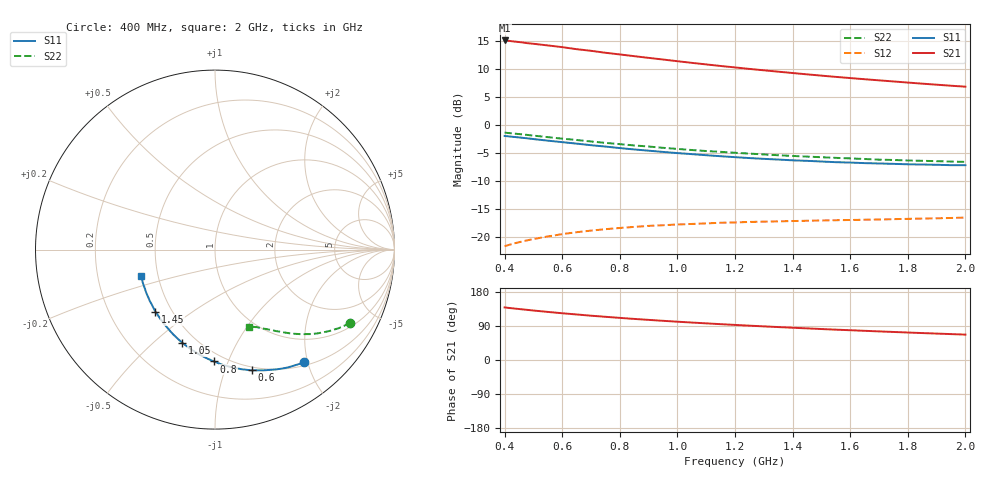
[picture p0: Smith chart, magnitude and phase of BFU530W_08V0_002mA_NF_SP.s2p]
! Filename:  P:\Prog\Test\Noise\ATS_data\Testdata_Net\06 Compressed Noise after Statistics\BFU530W_APM2013_09_A05_08p0V_002mA_NF_CM01_D.sf
! Date/Time: Tue 26/Mar/2013 18:06:04
! BFU530W_APM2013_09_A05_08p0V_1to25mA_NF_CM01_Bias2_R.sf
! Noise Parameter Data File
! BFU530W_APM2013_09_A05_08p0V_1to25mA_NF_CM01
! Date/time: Thu Mar 21 21:44:48 2013
! VAR V_out= 8.000000
! VAR I_out= 2.000000
! VAR V_in= 0.795400
! VAR I_in= 0.019805
! Device data file deembeded for feedlines and parallel
! Original file: \06 Compressed Noise after Statistics\BFU530W_APM2013_09_A05_08p0V_002mA_NF_CM01_R.sf
! Feed-files: PR019V01_070313_Feed1.s2p, PR019V01_070313_Feed2.s2p
! Parallel-file: PR019V01_070313_Par.s2p
# MHz S MA R 50
!  Freq-MHz  S11-mag  S11-arg  S21-mag  S21-arg  S12-mag  S12-arg  S22-mag  S22-arg
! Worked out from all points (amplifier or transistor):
!   37 points, 400 MHz to 2 GHz, reference 50 ohm
!   highest |S21| = 15.1 dB at 400 MHz (marker M1)
!   |S21| within 3 dB of that: start of sweep to 882.4 MHz
!   unconditionally stable (mu >= 1): nowhere
!   at 500 MHz: K = 0.28, MSG = 17.4 dB, |S12| = -20.3 dB
!   at 1.1 GHz: K = 0.57, MSG = 14.2 dB, |S12| = -17.5 dB
!   at 2 GHz: K = 0.94, MSG = 11.7 dB, |S12| = -16.5 dB
!   lowest NFmin = 0.46 dB at 420 MHz
!   S11 on the Smith chart (normalised r, x): 400 MHz: 0.55, -1.93; 600 MHz: 0.47, -1.24; 800 MHz: 0.44, -0.89; 1.05 GHz: 0.42, -0.62; 1.45 GHz: 0.41, -0.37; 2 GHz: 0.40, -0.15
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400  0.7996 -51.8  5.68 138.7  0.08308 60.5  0.8553 -28.4
420  0.7891 -54.2  5.616 136.9  0.086 59.4  0.8455 -29.5
440  0.7796 -56.4  5.536 135.3  0.08877 58.4  0.8355 -30.5
500  0.7497 -62.9  5.306 130.6  0.09616 55.4  0.8048 -33.4
550  0.7256 -68.0  5.129 126.9  0.1014 53.3  0.7796 -35.7
600  0.7034 -73.0  4.952 123.4  0.1064 51.3  0.7559 -37.7
650  0.6826 -77.5  4.749 120.2  0.1107 49.5  0.7352 -39.5
700  0.6609 -82.2  4.593 116.9  0.1143 47.9  0.7133 -41.3
750  0.6425 -86.4  4.411 114.0  0.1178 46.5  0.6935 -42.8
800  0.623 -90.7  4.263 111.2  0.1207 45.2  0.6754 -44.3
850  0.6056 -94.8  4.113 108.4  0.1234 44.1  0.6575 -45.6
950  0.5757 -102.3  3.84 103.4  0.1277 42.2  0.6262 -48.2
1050  0.5501 -109.4  3.586 98.8  0.1311 40.8  0.5986 -50.3
1150  0.527 -116.1  3.363 94.6  0.1343 39.7  0.5766 -52.2
1200  0.5169 -119.2  3.265 92.6  0.1353 39.4  0.5657 -53.3
1300  0.4993 -125.3  3.078 88.8  0.1374 38.8  0.5466 -55.1
1450  0.4793 -133.8  2.832 83.5  0.14 38.5  0.523 -57.6
1500  0.4727 -136.4  2.758 81.7  0.1409 38.5  0.5164 -58.5
1600  0.4626 -141.7  2.624 78.6  0.1422 38.8  0.5039 -60.1
1750  0.4506 -148.9  2.448 74.0  0.1447 39.7  0.488 -62.3
1850  0.4444 -153.6  2.34 71.1  0.1464 40.2  0.4798 -63.9
2000  0.4385 -160.2  2.198 67.0  0.1494 41.6  0.4692 -66.2
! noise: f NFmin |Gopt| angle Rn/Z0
400  0.4958  0.4958  24.31  0.1863
460  0.5083  0.4704  31.58  0.1842
600  0.5567  0.4903  37.23  0.1876
800  0.6057  0.4598  52.69  0.1646
1000  0.6852  0.4623  62.91  0.1654
1200  0.7307  0.4496  74.69  0.1527
1400  0.7386  0.4313  89.84  0.131
1600  0.7323  0.4158  102.6  0.1087
1800  0.893  0.4027  116.1  0.1016
2000  0.9471  0.394  129.5  0.0933
